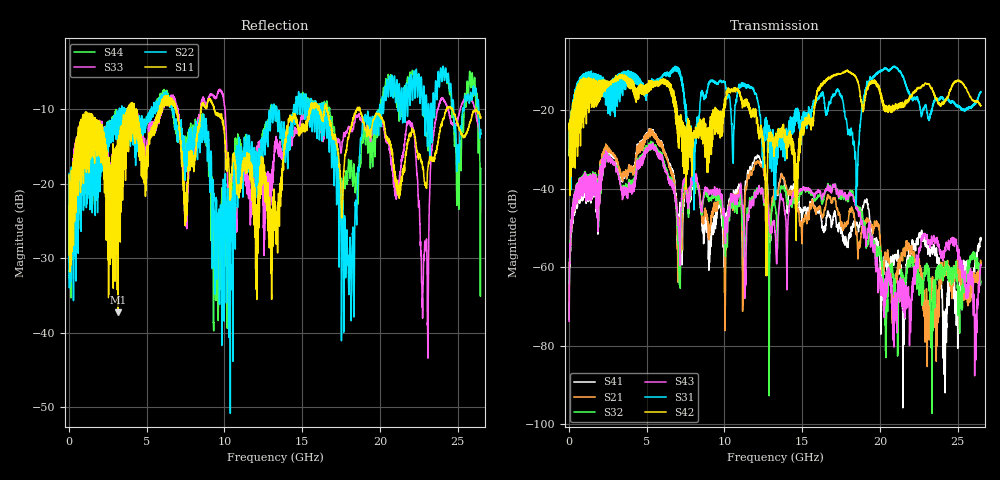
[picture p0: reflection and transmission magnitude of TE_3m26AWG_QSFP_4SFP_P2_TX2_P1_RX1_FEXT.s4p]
!Agilent Technologies,N5222A,MY51421691,A.10.00.00
!Agilent N5222A: A.10.00.00
!Date: Friday, January 30, 2015 12:36:24
!Correction: S11(Full 4 Port(1,2,3,4))
!S12(Full 4 Port(1,2,3,4))
!S13(Full 4 Port(1,2,3,4))
!S14(Full 4 Port(1,2,3,4))
!S21(Full 4 Port(1,2,3,4))
!S22(Full 4 Port(1,2,3,4))
!S23(Full 4 Port(1,2,3,4))
!S24(Full 4 Port(1,2,3,4))
!S31(Full 4 Port(1,2,3,4))
!S32(Full 4 Port(1,2,3,4))
!S33(Full 4 Port(1,2,3,4))
!S34(Full 4 Port(1,2,3,4))
!S41(Full 4 Port(1,2,3,4))
!S42(Full 4 Port(1,2,3,4))
!S43(Full 4 Port(1,2,3,4))
!S44(Full 4 Port(1,2,3,4))
!S4P File: Measurements: <S11,S12,S13,S14>,
!<S21,S22,S23,S24>,
!<S31,S32,S33,S34>,
!<S41,S42,S43,S44>:
# Hz S  dB  R 50.0
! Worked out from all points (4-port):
!   2650 points, 10 MHz to 26.5 GHz, reference 50 ohm
!   strongest paths, dB at 10 MHz, 6.63 GHz, 13.26 GHz, 19.88 GHz, 26.5 GHz:
!     S42: -24.9, -16.3, -29.6, -13.5, -18.9
!     S31: -24.9, -10.2, -30.3, -10.6, -15.3
!     S43: -73.8, -39.2, -50.8, -66.5, -59.5
!     S32: -63.6, -38.4, -44.3, -56.8, -63.6
!     S21: -67.2, -36.6, -40.3, -48.9, -59.0
!     S41: -73.3, -35.8, -40.7, -54.6, -53.2
!   lowest |S11| = -37.2 dB at 3.15 GHz (marker M1), VSWR 1.03, Z = 50.6 - j1.25 ohm
!   |S11| at or under -10 dB: start of sweep to 3.77 GHz; 9.336 GHz to 15.5 GHz (6.16 GHz wide, 49.6 % of centre); 18.72 GHz to 24.29 GHz (5.571 GHz wide, 25.9 % of centre)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
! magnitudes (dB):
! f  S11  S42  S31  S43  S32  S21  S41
! 10 MHz  -18.8  -24.9  -24.9  -73.8  -63.6  -67.2  -73.3
! 3.15 GHz  -37.2  -12.5  -16.9  -35.8  -35.7  -33.6  -34.3
! 12.68 GHz  -19.1  -45.5  -21.9  -44.5  -45.5  -38.1  -37.4
! 18.08 GHz  -13.0  -10.4  -26.5  -41.0  -40.4  -45.1  -51.2
! 20.96 GHz  -18.7  -19.7  -8.8  -73.7  -63.5  -68.9  -57.5
! 24.18 GHz  -10.6  -17.7  -17.3  -54.9  -59.9  -61.6  -74.3
! 26.5 GHz  -11.1  -18.9  -15.3  -59.5  -63.6  -59.0  -53.2
